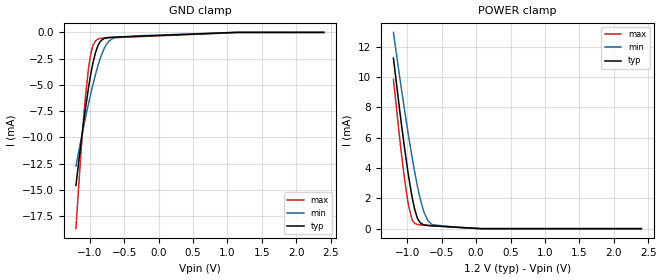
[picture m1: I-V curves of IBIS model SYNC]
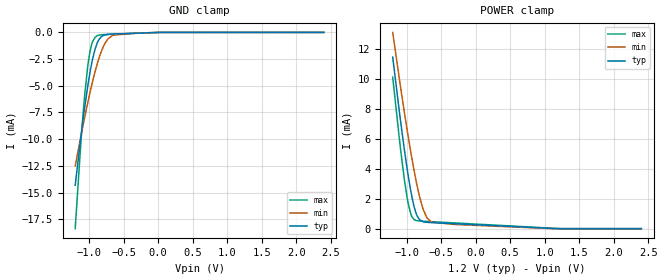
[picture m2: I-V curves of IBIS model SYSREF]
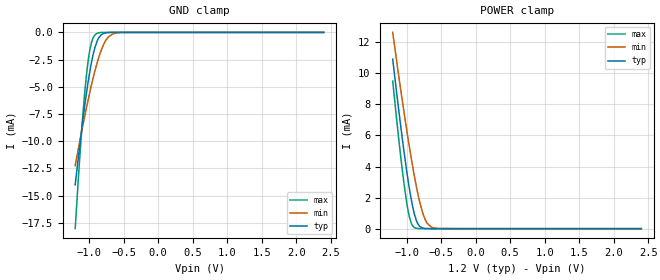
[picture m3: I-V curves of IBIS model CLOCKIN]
| Texas Instruments Incorporated
| Low-Noise Clock Jitter Cleaner with Dual Loop PLLs
| Marketing part#   Voltage Range   Package-type   #pins/pkg drawing
| ADC131JB68RTA   1.15V - 1.25V   QFN   40
[IBIS Ver]   4.1
[File name]   adc31jb68.ibs
[File Rev]   1.0
[Date]   09/09/2015
[Source]   Model built from spectre simulations at:
   Texas Instruments Incorporated.
   Analog-eLab, HPA
   12500 TI Blvd
   Dallas, TX -75243
   For Support e-mail: elab_ibis@list.ti.com
[Notes]   Revision History
   Rev 1.0: 09/09/2015
   - ccomp values are based on PVT settings:
   MIN: Low Voltage, High Temperature, Weak Process
   TYP: Nominal Voltage, Nominal Temperature, Nominal Process
   MAX: High Voltage, Low Temperature, Fast Process
   - C_comp although listed in numerical order of value are obtained from varying PVT conditions.
   For PVT conditions for each specific value, refer to the buffer description under respective [Model].
   IBIS model user is responsible for using appropriate C_comp to simulate for Signal Integrity.
   - On chip termination is provided for CLKIN, SYSREF and SYNC differential input buffers.
   Some simulators will show fewer reflections and cleaner signals if the Series Pin Mapping
   is disabled (commented out) and an external terminating resistor is added to the schematic.
   For the CLKIN, SYSREF, and SYNCb inputs, a 100 Ohm terminating resistor should be used.
   - SDO Pullup and Pulldown non-monotonic in behavior
[Disclaimer]  This model is designed as an aid for customers of Texas Instruments
 TI and its licensors and suppliers make no warranties, either expressed
 or implied, with respect to this  model, including the warranties of
 merchantability or fitness for a particular purpose.
 The model is provided solely on an "as is" basis. The entire risk as to
 its quality and performance is with the customer.
[Copyright] (C)Copyright 2015 Texas Instruments Incorporated.
   All rights reserved.
[Component]   ADC31JB68RTA
[Manufacturer]  Texas Instruments Incorporated
[Package]   |40-pin QFN package
|   typ   min   max
R_pkg   0.0514   0.0060   0.1075
L_pkg   0.9640n   0.1132n   1.5124n
C_pkg   0.3870p   0.2258p   1.4002p
[Pin]   signal_name   model_name   R_pin   L_pin   C_pin
1   VA3.0   NC   0.00600  0.11317n  1.40017p
2   VA3.0   NC   0.03089  0.84634n  0.46274p
3   AGND   NC   0.02856  0.72934n  0.43520p
4   VINBM   NC   0.03921  0.73222n  0.28457p
5   VINBP   NC   0.03837  0.70763n  0.37479p
6   AGND   NC   0.02708  0.66269n  0.29708p
7   VCM   NC   0.04096  0.77938n  0.39666p
8   VACLK1.2   NC   0.03096  0.83534n  0.34055p
9   VACLK1.2   NC   0.03330  0.96058n  0.46407p
10   AGND   NC   0.03505  1.09989n  0.30927p
11   CLKINP   CLOCKIN   0.04905  1.04876n  0.49014p
12   CLKINN   CLOCKIN   0.04373  0.85845n  0.32601p
13   AGND   NC   0.04223  0.80461n  0.41499p
14   AGND   NC   0.04197  0.78737n  0.30017p
15   VA1.8   POWER   0.03065  0.83050n  0.43113p
16   VA1.8   POWER   0.03106  0.80939n  0.33026p
17   SYSREFP   SYSREF   0.09189  1.26434n  0.38448p
18   SYSREFN   SYSREF   0.10749  1.51244n  0.30570p
19   SYNCbP   SYNC   0.08612  1.17341n  0.27203p
20   SYNCbN   SYNC   0.09442  1.30819n  0.22580p
21   VA1.2   NC   0.03608  1.12283n  0.52672p
22   AGND   NC   0.04861  0.98996n  0.34267p
23   SO1P   NC   0.09083  1.24927n  0.38666p
24   SO1N   NC   0.08396  1.14184n  0.25944p
25   SO0P   NC   0.08290  1.12513n  0.35082p
26   SO0N   NC   0.08785  1.20233n  0.25738p
27   AGND   NC   0.03280  0.90151n  0.45173p
28   VA1.8   POWER   0.03493  1.01620n  0.38152p
29   VA1.2   NC   0.03569  1.02090n  0.49260p
30   AGND   NC   0.03519  1.07775n  0.30372p
31   CSB   SDI   0.09465  1.31195n  0.45949p
32   SCLK   SDI   0.08566  1.16634n  0.28597p
33   SDI   SDI   0.08122  1.09457n  0.37152p
34   SDO   SDO   0.08421  1.13961n  0.26261p
35   VA1.2   NC   0.02967  0.76879n  0.40839p
36   VA1.2   NC   0.02987  0.77825n  0.30944p
37   AGND   NC   0.04368  0.83080n  0.42645p
38   AGND   NC   0.04409  0.85699n  0.32409p
39   VA1.8   NC   0.03148  0.84377n  0.34738p
40   VA1.8   NC   0.03429  1.05699n  0.28664p
[Diff pin]  inv_pin  vdiff  tdelay_typ  tdelay_min  tdelay_max
11   12   0.0   0.0s   0.0s   0.0s
17   18   0.0   0.0s   0.0s   0.0s
19   20   0.0   0.0s   0.0s   0.0s
[Series Pin Mapping] pin_2 model_name function_table_group
11   12   100_ohm
17   18   100_ohm
19   20   100_ohm
[Model]   100_ohm
Model_type   Series
|   typ   min   max
C_comp   0   0   0
[Voltage Range]   1.8   1.7   1.9
[Temperature Range]   27   125   -40
[R series]   100   94   106
| Models and submodels in the file (6): SYNC (Input), SYSREF (Input), CLOCKIN (Input), SDI (Input), SDO (Output), 100_ohm (Series)
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|   Model SYNC
[Model]   SYNC
Model_type   Input
Vinl = 0.4
Vinh = 0.75
|   typ   min   max
C_comp   0.1841pF   0.1807pF   0.1863pF
[Voltage Range]   1.2   1.15   1.25
[Temperature Range]   27   125   -40
[Power Clamp Reference]   1.2   1.15   1.25
[GND Clamp Reference]   0   0   0
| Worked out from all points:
|   GND clamp passes 1 mA (typ) near -0.86 V on its own axis
|   POWER clamp passes 1 mA (typ) near -0.87 V on its own axis
[GND Clamp]
|   Voltage   I(typ)   I(min)   I(max)
-1.2V     -14.58mA   -12.72mA   -18.68mA
-1.124V   -10.41mA   -10.17mA   -11.24mA
-1.06V    -7.161mA   -8.082mA   -5.975mA
-1.016V   -5.237mA   -6.765mA   -3.386mA
-984mV    -3.966mA   -5.823mA   -2.059mA
-951.6mV  -2.879mA   -4.93mA    -1.25mA
-915.6mV  -1.924mA   -4.005mA   -810uA
-858mV    -984.1uA   -2.707mA   -587uA
-782.4mV  -559.9uA   -1.44mA    -537.2uA
-649.2mV  -450uA     -514.9uA   -501.3uA
1.075V    -14.5uA    -588.2nA   -29.79uA
2.4V      0A         0A         0A
[POWER Clamp]
|   Voltage   I(typ)   I(min)   I(max)
-1.2V     11.25mA    12.96mA    9.858mA
-1.106V   7.716mA    9.938mA    5.858mA
-1.034V   5.191mA    7.718mA    3.144mA
-987.6mV  3.697mA    6.34mA     1.717mA
-937.2mV  2.291mA    4.934mA    710.9uA
-894mV    1.334mA    3.813mA    365.6uA
-854.4mV  732.4uA    2.874mA    279.1uA
-764.4mV  258.9uA    1.199mA    234.7uA
-703.2mV  210.2uA    550.9uA    217uA
-638.4mV  188.2uA    266uA      198.7uA
70.8mV    321.6nA    392nA      157.8nA
2.4V      0A         0A         0A
|   Model SYSREF
[Model]   SYSREF
Model_type   Input
Vinl = 0.5
Vinh = 0.75
|   typ   min   max
C_comp   0.2493p   0.2133p   0.2765p
[Voltage Range]   1.2   1.15   1.25
[Temperature Range]   27   125   -40
[Power Clamp Reference]   1.2   1.15   1.25
[GND Clamp Reference]   0   0   0
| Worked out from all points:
|   GND clamp passes 1 mA (typ) near -0.88 V on its own axis
|   POWER clamp passes 1 mA (typ) near -0.86 V on its own axis
[GND Clamp]
|   Voltage   I(typ)   I(min)   I(max)
-1.2V     -14.31mA   -12.51mA   -18.38mA
-1.124V   -10.13mA   -9.943mA   -10.92mA
-1.099V   -8.825mA   -9.116mA   -8.717mA
-1.06V    -6.878mA   -7.85mA    -5.658mA
-1.016V   -4.951mA   -6.527mA   -3.066mA
-984mV    -3.678mA   -5.582mA   -1.738mA
-958.8mV  -2.813mA   -4.88mA    -1.067mA
-883.2mV  -1.016mA   -2.993mA   -318.3uA
-829.2mV  -451.9uA   -1.906mA   -228.9uA
-764.4mV  -227uA     -965.8uA   -201.7uA
-649.2mV  -151.2uA   -254.2uA   -169.2uA
2.4V      0A         0A         0A
[POWER Clamp]
|   Voltage   I(typ)   I(min)   I(max)
-1.2V     11.44mA    13.09mA    10.11mA
-1.106V   7.91mA     10.08mA    6.109mA
-1.034V   5.388mA    7.862mA    3.398mA
-987.6mV  3.896mA    6.487mA    1.972mA
-937.2mV  2.492mA    5.084mA    968uA
-894mV    1.538mA    3.966mA    624.1uA
-854.4mV  937.9uA    3.029mA    538.9uA
-764.4mV  468.5uA    1.359mA    497.5uA
-703.2mV  422.5uA    714.5uA    481.9uA
-638.4mV  403.4uA    433.2uA    465.7uA
1.126V    11.81uA    232.2nA    25.91uA
2.4V      0A         0A         0A
|   Model CLOCKIN
[Model]   CLOCKIN
Model_type   Input
Vinl = 0.5
Vinh = 0.75
|   typ   min   max
C_comp   0.2493p   0.2133p   0.2765p
[Voltage Range]   1.2   1.15   1.25
[Temperature Range]   27   125   -40
[Power Clamp Reference]   1.2   1.15   1.25
[GND Clamp Reference]   0   0   0
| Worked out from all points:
|   GND clamp passes 1 mA (typ) near -0.89 V on its own axis
|   POWER clamp passes 1 mA (typ) near -0.89 V on its own axis
[GND Clamp]
|   Voltage   I(typ)   I(min)   I(max)
-1.2V     -14.01mA   -12.25mA   -18.04mA
-1.146V   -11.01mA   -10.42mA   -12.62mA
-1.099V   -8.557mA   -8.879mA   -8.414mA
-1.067V   -6.962mA   -7.849mA   -5.878mA
-1.034V   -5.475mA   -6.85mA    -3.755mA
-980.4mV  -3.312mA   -5.273mA   -1.357mA
-951.6mV  -2.362mA   -4.485mA   -670uA
-915.6mV  -1.414mA   -3.565mA   -239.2uA
-858mV    -487.4uA   -2.276mA   -31.05uA
-782.4mV  -80.24uA   -1.022mA   -950.5nA
-645.6mV  -778.7nA   -113.1uA   -19.21nA
2.4V      0A         0A         0A
[POWER Clamp]
|   Voltage   I(typ)   I(min)   I(max)
-1.2V     10.91mA    12.64mA    9.501mA
-1.124V   8.06mA     10.21mA    6.26mA
-1.052V   5.502mA    7.981mA    3.462mA
-994.8mV  3.634mA    6.281mA    1.612mA
-951.6mV  2.394mA    5.071mA    641.7uA
-922.8mV  1.678mA    4.302mA    270.4uA
-894mV    1.078mA    3.572mA    94.68uA
-840mV    343.8uA    2.331mA    10.69uA
-804mV    127.3uA    1.625mA    2.327uA
-732mV    13.47uA    602uA      85.41nA
-638.4mV  575nA      89.3uA     692.6pA
2.4V      0A         0A         0A
